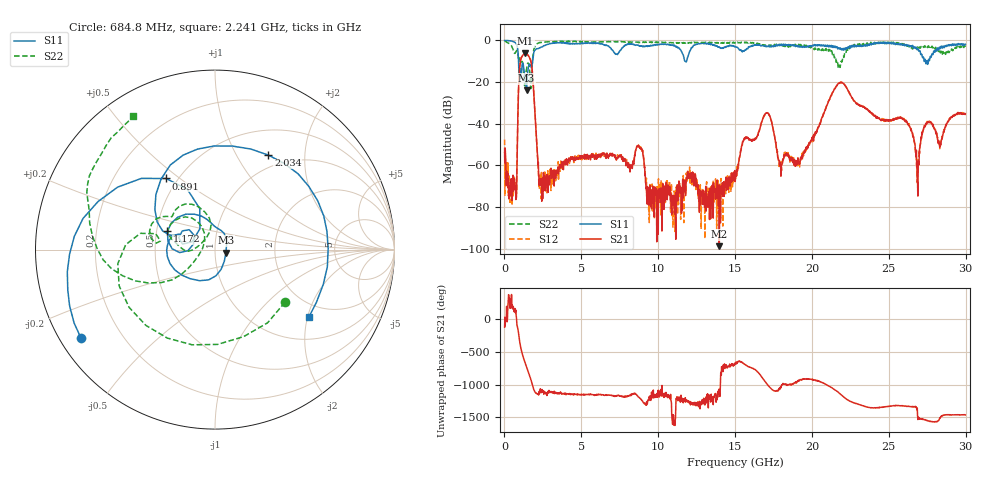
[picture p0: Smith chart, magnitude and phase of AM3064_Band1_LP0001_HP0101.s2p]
# Hz S DB R 50.0
!freq dBS11 angS11 dBS21 angS21 dBS12 angS12 dBS22 angS22
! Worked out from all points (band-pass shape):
!   1600 points, 10 MHz to 29.98 GHz, reference 50 ohm
!   highest |S21| = -6.23 dB at 1.36 GHz (marker M1); lowest = -98.8 dB at 13.97 GHz (marker M2)
!   |S21| within 3 dB of the highest: 1.061 GHz to 1.688 GHz (627 MHz wide, 45.6 % of centre)
!   lowest |S11| = -24.0 dB at 1.435 GHz (marker M3), VSWR 1.14, Z = 56.5 - j1.84 ohm
!   |S11| at or under -10 dB: 916.6 MHz to 1.831 GHz (914.2 MHz wide, 66.5 % of centre); 11.74 GHz to 11.84 GHz (100.6 MHz wide, 0.853 % of centre); 27.39223 GHz to 27.46086 GHz (68.63 MHz wide, 0.25 % of centre)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
!   |S22| runs from -23.1 to -0.2 dB; largest |S21 - S12| = 0.0055
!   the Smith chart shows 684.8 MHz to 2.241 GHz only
!   S11 on the Smith chart (normalised r, x): 684.8 MHz: 0.06, -0.30; 891 MHz: 0.43, +0.45; 1.172 GHz: 0.57, +0.13; 2.034 GHz: 0.82, +1.37; 2.241 GHz: 1.59, -2.04
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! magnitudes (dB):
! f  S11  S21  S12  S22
! 10 MHz  0.0  -53.9  -47.5  -0.2
! 684.8 MHz  -1.0  -70.1  -71.9  -6.2
! 891 MHz  -6.4  -30.3  -30.3  -7.4
! 1.172 GHz  -10.9  -7.4  -7.3  -10.4
! 1.36 GHz  -19.0  -6.2  -6.2  -18.2
! 1.435 GHz  -24.0  -6.4  -6.4  -13.9
! 1.753 GHz  -13.3  -11.2  -11.2  -17.2
! 2.034 GHz  -4.4  -41.1  -41.2  -2.1
! 2.241 GHz  -3.8  -65.5  -70.3  -1.2
! 5.015 GHz  -1.3  -56.5  -56.1  -0.7
! 8.763 GHz  -2.8  -50.9  -50.8  -1.1
! 10 GHz  -2.0  -93.0  -68.3  -0.9
! 13.97 GHz  -3.3  -98.8  -80.0  -1.1
! 15 GHz  -3.0  -67.8  -63.3  -1.3
! 17.03 GHz  -3.0  -34.7  -34.8  -2.6
! 17.95 GHz  -2.3  -60.2  -59.4  -2.1
! 19.99 GHz  -2.9  -47.9  -47.9  -3.4
! 21.83 GHz  -3.8  -20.3  -20.3  -13.0
! 25 GHz  -1.0  -38.1  -38.2  -1.1
! 26.87 GHz  -4.4  -68.5  -57.2  -3.3
! 27.43 GHz  -11.2  -39.8  -39.7  -2.9
! 29.98 GHz  -1.8  -35.2  -35.3  -3.1
